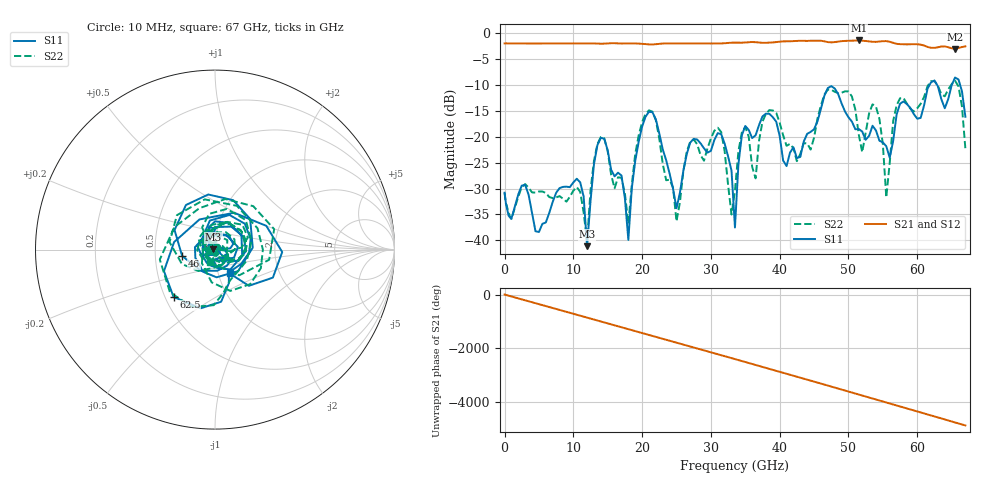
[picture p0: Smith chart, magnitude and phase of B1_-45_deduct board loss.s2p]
!Keysight Technologies,N5247B,MY61255065,A.16.20.04
!Date: Sunday, September 03, 2023 21:42:04
!Correction: S11(C  2-Port  )
!S21(C  2-Port  )
!S12(C  2-Port  )
!S22(C  2-Port  )
!S2P File: Measurements: S11, S21, S12, S22:
!Deduct Board Loss
# Hz S  dB  R 50
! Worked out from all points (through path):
!   142 points, 10 MHz to 67 GHz, reference 50 ohm
!   highest |S21| = -1.37 dB at 51.5 GHz (marker M1); lowest = -3.0 dB at 65.5 GHz (marker M2)
!   lowest |S11| = -41.1 dB at 12 GHz (marker M3), VSWR 1.02, Z = 49.1 + j0.0673 ohm
!   |S11| at or under -10 dB: start of sweep to 61.78 GHz; 62.9 GHz to 65.01 GHz (2.108 GHz wide, 3.3 % of centre); 66.24 GHz to end of sweep
!   |S22| runs from -40.3 to -9.1 dB; largest |S21 - S12| = 0.0026
!   S11 on the Smith chart (normalised r, x): 10 MHz: 0.94, -0.00; 46 GHz: 0.69, -0.05; 62.5 GHz: 0.55, -0.33; 67 GHz: 1.13, -0.31
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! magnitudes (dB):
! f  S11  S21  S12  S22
! 10 MHz  -30.8  -1.9  -1.9  -30.8
! 11.5 GHz  -31.5  -1.9  -1.9  -34.6
! 12 GHz  -41.1  -1.9  -1.9  -40.3
! 14 GHz  -20.2  -2.0  -2.0  -20.0
! 18 GHz  -39.9  -1.9  -1.9  -36.8
! 20 GHz  -18.0  -2.0  -2.0  -17.2
! 22.5 GHz  -19.3  -2.0  -2.0  -20.4
! 25 GHz  -33.8  -1.9  -1.9  -36.3
! 27 GHz  -21.1  -2.0  -2.0  -20.9
! 31.5 GHz  -19.5  -1.9  -1.9  -19.1
! 33 GHz  -26.5  -1.8  -1.8  -35.0
! 33.5 GHz  -37.5  -1.8  -1.8  -30.4
! 34 GHz  -25.4  -1.8  -1.8  -22.8
! 45 GHz  -18.5  -1.4  -1.4  -20.1
! 46 GHz  -14.6  -1.4  -1.4  -13.9
! 51.5 GHz  -18.5  -1.4  -1.4  -19.6
! 54 GHz  -18.8  -1.6  -1.6  -14.2
! 56 GHz  -24.0  -1.6  -1.6  -25.0
! 57.5 GHz  -13.6  -2.1  -2.1  -12.5
! 62.5 GHz  -9.1  -2.8  -2.8  -9.2
! 65.5 GHz  -8.5  -3.0  -3.0  -9.1
! 67 GHz  -16.1  -2.5  -2.5  -22.3
